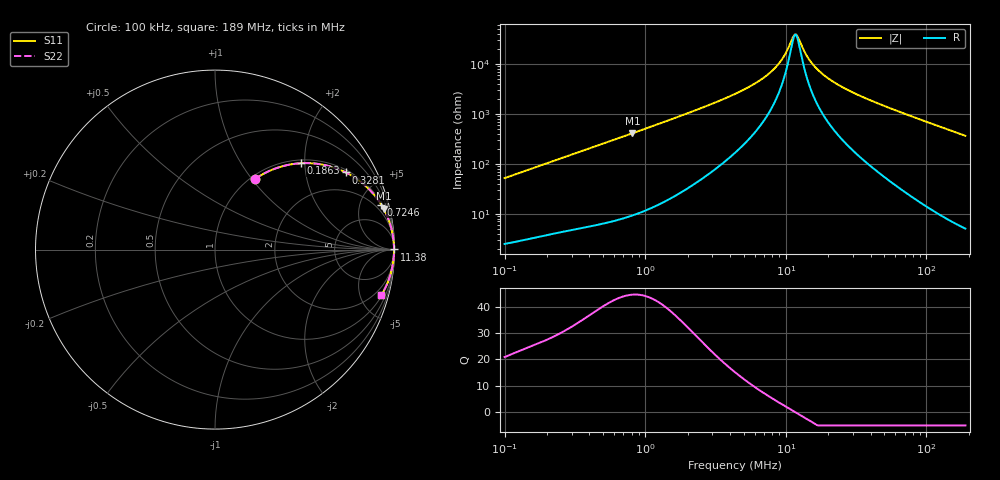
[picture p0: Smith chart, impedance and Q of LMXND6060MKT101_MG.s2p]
! LMXND6060MKT101_MG  S-PARAMETER MODEL  ( General Type )
! Model Generated by TAIYO YUDEN Corporation (https://www.yuden.co.jp/en/)
! Version 1.0
! TAIYO YUDEN Control No. 191025NI43SB-FBB
! Copyright(c) 2019 TAIYO YUDEN CO.,LTD. All Rights Reserved.
! Product Description (link to TY-COMPAS)
! https://ds.yuden.co.jp/TYCOMPAS/or/detail?pn=LMXND6060MKT101MMG&u=M
! Products Name : Inductors
! Characteristics :
!  Inductance : 100 uH , SRF(min) : 1.0 MHz , DC Resistance(max) : 2.004 Ohm
!  Rated Current : Saturation :350 mA , Temp Rise : 320 mA (40 degC)
!  Case Size : 6.0 x 6.0 / 0.236 x 0.236 [mm/inch] , Thickness : 1.2 / 0.047 [mm/inch]
!  (Conditions: Temperature = 25 degC , DC Bias Current/Voltage = 0A / 0V)
! External Node Assignments :
!  1  o---GGG---o  2
! GND o---------o GND
! Frequency Range : 0.1MHz  -  189.042664MHz  [ 402 STEP ]
# MHz S RI R 50
! Freq[MHz].  S11 Real  S11 Imag  S21 Real  S21 Imag  S12 Real  S12 Imag  S22 Real  S22 Imag
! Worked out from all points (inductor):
!   401 points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, 100 kHz to 189 MHz, reference 50 ohm
!   read as one part in series: L = 82 uH near 103.8 kHz
!   highest Q = 44.6 at 811.4 kHz (marker M1), where L = 80.5 uH
!   self-resonance near 11.59 MHz
!   S11 on the Smith chart (normalised r, x): 100 kHz: 1.05, +1.03; 186.3 kHz: 1.07, +1.91; 328.1 kHz: 1.10, +3.33; 724.6 kHz: 1.17, +7.33; 11.38 MHz: open; 189 MHz: 1.10, -7.32
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0.1  0.222 0.3924  0.778 -0.3924  0.778 -0.3924  0.222 0.3924
0.186344  0.4778 0.4812  0.5222 -0.4812  0.5222 -0.4812  0.4778 0.4812
0.328139  0.7293 0.4297  0.2707 -0.4297  0.2707 -0.4297  0.7293 0.4297
0.353854  0.757 0.4148  0.243 -0.4148  0.243 -0.4148  0.757 0.4148
0.4969  0.8573 0.3375  0.1427 -0.3375  0.1427 -0.3375  0.8573 0.3375
0.724598  0.9258 0.2509  0.0742 -0.2509  0.0742 -0.2509  0.9258 0.2509
0.811419  0.9395 0.2275  0.0605 -0.2275  0.0605 -0.2275  0.9395 0.2275
1.252125  0.9725 0.152  0.0275 -0.152  0.0275 -0.152  0.9725 0.152
4.347904  0.9959 0.0392  0.00413 -0.0392  0.00413 -0.0392  0.9959 0.0392
6.221807  0.9969 0.0228  0.00306 -0.0228  0.00306 -0.0228  0.9969 0.0228
8.102072  0.9973 0.0127  0.00268 -0.0127  0.00268 -0.0127  0.9973 0.0127
9.601049  0.9974 0.00675  0.00255 -0.00675  0.00255 -0.00675  0.9974 0.00675
11.37735  0.9975 0.000964  0.00251 -0.000964  0.00251 -0.000964  0.9975 0.000964
12.0397  0.9975 -0.000949  0.0025 0.000949  0.0025 0.000949  0.9975 -0.000949
13.73901  0.9975 -0.00544  0.00253 0.00544  0.00253 0.00544  0.9975 -0.00544
15.38522  0.9974 -0.00935  0.00259 0.00935  0.00259 0.00935  0.9974 -0.00935
18.5788  0.9972 -0.0162  0.00276 0.0162  0.00276 0.0162  0.9972 -0.0162
23.74138  0.9968 -0.0259  0.00318 0.0259  0.00318 0.0259  0.9968 -0.0259
33.33888  0.9957 -0.0421  0.00431 0.0421  0.00431 0.0421  0.9957 -0.0421
54.44117  0.9918 -0.0745  0.00819 0.0745  0.00819 0.0745  0.9918 -0.0745
103.3796  0.9759 -0.1441  0.0241 0.1441  0.0241 0.1441  0.9759 -0.1441
189.0427  0.9275 -0.2525  0.0725 0.2525  0.0725 0.2525  0.9275 -0.2525
